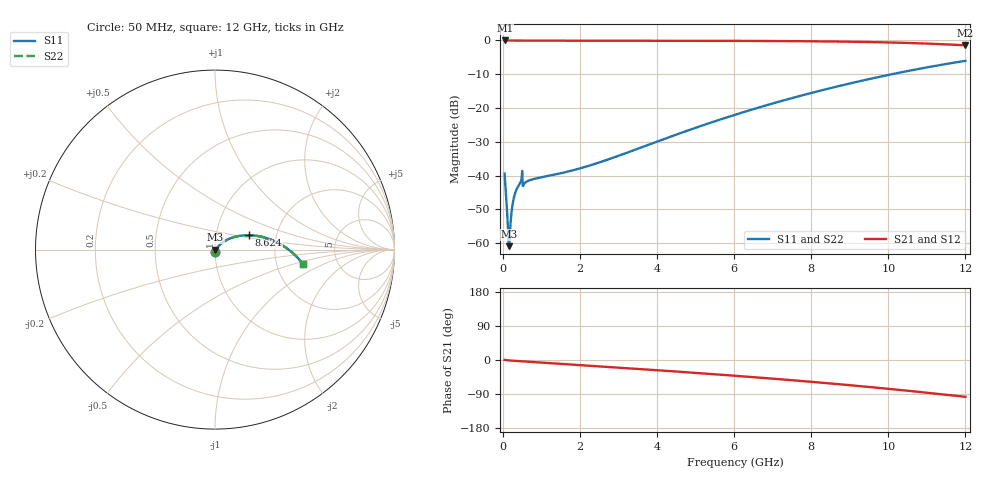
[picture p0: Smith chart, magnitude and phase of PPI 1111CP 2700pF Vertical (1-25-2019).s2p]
# GHz S MA R 50
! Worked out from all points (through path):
!   1601 points, 50 MHz to 12 GHz, reference 50 ohm
!   highest |S21| = 0.00 dB at 57.47 MHz (marker M1); lowest = -1.4 dB at 12 GHz (marker M2)
!   group delay of S21, straight-line fit = 22 ps
!   lowest |S11| = -60.9 dB at 162 MHz (marker M3), VSWR 1.00, Z = 50.1 - j0.0315 ohm
!   |S11| at or under -10 dB: start of sweep to 10.09 GHz
!   |S22| runs from -60.9 to -6.0 dB; largest |S21 - S12| = 0
!   S11 on the Smith chart (normalised r, x): 50 MHz: 1.00, -0.02; 8.624 GHz: 1.44, +0.24; 12 GHz: 2.84, -0.62
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0.05  0.01072 -87.7  0.9996 0.3  0.9996 0.3  0.01072 -87.7
0.05746875  0.00908 -87.4  0.9996 0.2  0.9996 0.2  0.00908 -87.4
0.079875  0.005832 -85.9  0.9995 -0.2  0.9995 -0.2  0.005832 -85.9
0.1246875  0.002319 -76.2  0.9994 -0.7  0.9994 -0.7  0.002319 -76.2
0.139625  0.001553 -65.3  0.9993 -0.8  0.9993 -0.8  0.001553 -65.3
0.1620312  0.0009063 -20.3  0.9991 -1.0  0.9991 -1.0  0.0009063 -20.3
0.1844375  0.001291 29.4  0.9989 -1.2  0.9989 -1.2  0.001291 29.4
0.199375  0.001802 41.5  0.9987 -1.3  0.9987 -1.3  0.001802 41.5
0.259125  0.003837 49.4  0.9976 -1.8  0.9976 -1.8  0.003837 49.4
0.3039375  0.005074 46.9  0.9967 -2.2  0.9967 -2.2  0.005074 46.9
0.3562187  0.006196 43.0  0.9956 -2.5  0.9956 -2.5  0.006196 43.0
0.4533125  0.007792 37.5  0.994 -3.2  0.994 -3.2  0.007792 37.5
0.5802812  0.007863 28.4  0.9933 -4.0  0.9933 -4.0  0.007863 28.4
0.796875  0.008897 26.2  0.9924 -5.4  0.9924 -5.4  0.008897 26.2
2.044156  0.013 33.8  0.991 -13.6  0.991 -13.6  0.013 33.8
4.038312  0.03244 45.1  0.9894 -27.1  0.9894 -27.1  0.03244 45.1
6.025  0.07952 40.2  0.9852 -41.6  0.9852 -41.6  0.07952 40.2
8.019156  0.1682 27.7  0.9719 -57.7  0.9719 -57.7  0.1682 27.7
8.624125  0.2052 23.0  0.9641 -63.0  0.9641 -63.0  0.2052 23.0
10.01331  0.3099 10.8  0.9342 -76.2  0.9342 -76.2  0.3099 10.8
11.00666  0.4 1.1  0.8984 -86.4  0.8984 -86.4  0.4 1.1
12  0.4991 -9.4  0.8468 -97.2  0.8468 -97.2  0.4991 -9.4
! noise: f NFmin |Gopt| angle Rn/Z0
0.05  0.0004222  0.881  0.3252  0.0007681
1.372  0.01038  0.8687  8.76  0.0169
2.701  0.01514  0.8291  17.13  0.01824
4.031  0.01905  0.8048  25.27  0.01931
5.36  0.02267  0.7904  33.13  0.0205
6.682  0.02622  0.7835  40.58  0.02192
8.012  0.0299  0.7826  47.68  0.02368
9.341  0.03385  0.7865  54.37  0.0259
10.67  0.03823  0.7946  60.64  0.02877
12  0.04331  0.8062  66.51  0.03267
